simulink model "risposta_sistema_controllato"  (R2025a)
settings: Solver=VariableStepAuto  StartTime=0.0  StopTime=10  RelTol=1e-3
undefined symbols (not defined in the file): denCs, denGs, K, numCs, numGs

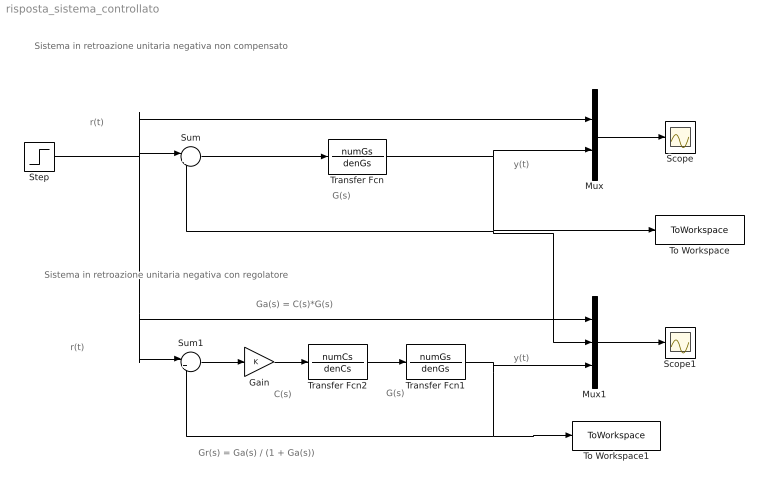
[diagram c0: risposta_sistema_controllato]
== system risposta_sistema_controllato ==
  note: Gr(s) = Ga(s) / (1 + Ga(s))
  note: Ga(s) = C(s)*G(s)
  note: C(s)
  note: Sistema in retroazione unitaria negativa non compensato
  note: y(t)
  note: r(t)
  note: G(s)
  note: Sistema in retroazione unitaria negativa con regolatore
  note: G(s)
  note: r(t)
  note: y(t)
  Gain : Gain  Gain=K
  Mux : Mux  Inputs=2
  Mux1 : Mux  Inputs=3
  Scope : Scope
  Scope1 : Scope
  Step : Step  Time=0  SampleTime=0
  Sum : Sum  Inputs=|+-
  Sum1 : Sum  Inputs=|+-
  To Workspace : ToWorkspace  VariableName=ync  SampleTime=-1
  To Workspace1 : ToWorkspace  VariableName=yc  SampleTime=-1
  Transfer Fcn : TransferFcn  Numerator=numGs  Denominator=denGs
  Transfer Fcn1 : TransferFcn  Numerator=numGs  Denominator=denGs
  Transfer Fcn2 : TransferFcn  Numerator=numCs  Denominator=denCs
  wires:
  Sum/1 -> Transfer Fcn/1
  Transfer Fcn/1 -> Mux/2, Mux1/2, Sum/2, To Workspace/1
  Mux/1 -> Scope/1
  Mux1/1 -> Scope1/1
  Transfer Fcn1/1 -> Mux1/3, To Workspace1/1, Sum1/2
  Transfer Fcn2/1 -> Transfer Fcn1/1
  Sum1/1 -> Gain/1
  Gain/1 -> Transfer Fcn2/1
  Step/1 -> Sum1/1, Mux1/1, Mux/1, Sum/1
